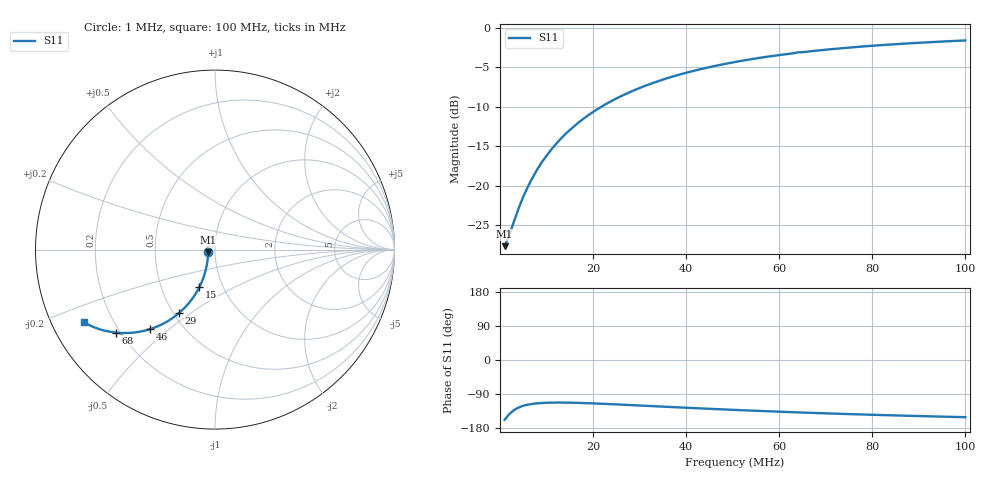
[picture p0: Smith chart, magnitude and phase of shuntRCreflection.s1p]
# Hz S RI R 50.0
! written by SimSmith version 18.3b
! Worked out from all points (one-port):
!   100 points, 1 MHz to 100 MHz, reference 50 ohm
!   lowest |S11| = -27.7 dB at 1 MHz (marker M1), VSWR 1.09, Z = 46.3 - j1.44 ohm
!   |S11| at or under -10 dB: start of sweep to 21.78 MHz
!   S11 on the Smith chart (normalised r, x): 1 MHz: 0.93, -0.03; 15 MHz: 0.78, -0.34; 29 MHz: 0.54, -0.45; 46 MHz: 0.33, -0.43; 68 MHz: 0.18, -0.35; 100 MHz: 0.10, -0.26
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1000000  -0.0381 -0.0155
2000000  -0.0384 -0.0292
4000000  -0.0414 -0.0583
5000000  -0.0433 -0.0729
6000000  -0.0458 -0.087
7000000  -0.0489 -0.1007
8000000  -0.052 -0.1152
9000000  -0.0561 -0.1291
1e7  -0.0599 -0.1422
1.2e7  -0.0696 -0.1693
1.4e7  -0.081 -0.1953
1.5e7  -0.0865 -0.2078
1.7e7  -0.0999 -0.2323
2e7  -0.1214 -0.2669
2.3e7  -0.1458 -0.2985
2.6e7  -0.1717 -0.3267
2.9e7  -0.1993 -0.3522
3.4e7  -0.2468 -0.3881
3.9e7  -0.2957 -0.4163
4.6e7  -0.3635 -0.4434
5.1e7  -0.4101 -0.4556
5.7e7  -0.4633 -0.4633
6.3e7  -0.5121 -0.4646
6.4e7  -0.523 -0.4678
6.8e7  -0.5501 -0.4627
7.6e7  -0.6044 -0.4541
8.8e7  -0.6732 -0.4324
1e8  -0.7291 -0.406
